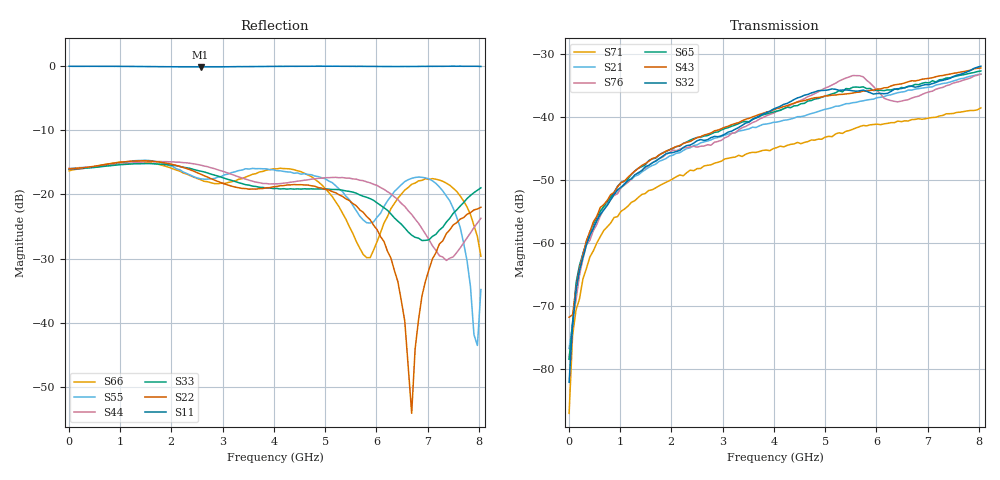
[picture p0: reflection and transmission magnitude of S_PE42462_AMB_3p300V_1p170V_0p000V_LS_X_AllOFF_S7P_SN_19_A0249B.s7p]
! Device ID: PE42462
! File Path: z:\PE42462\DataSheet S-parameter-6T\With_All_Off_States\Remeasure\AMB\3p300\LS_X\PE42462_AMB_3p300V_1p170V_0p000V_LS_X_AllOFF_S7P_SN_19_A0249B.s7p
! Serial: 19
! Lot: A0249B
! Temp: AMB
! VDD: 3.300
! VSS: 0.000
! Control_Hi: 1.170
! Control_Lo: 0.000
! Logic State: LS_X_AllOFF
! Port 1:
! Port 2:
! Port 3:
! Port 4:
! Port 5:
! Port 6:
! Port 7:
! ThroughPath:1-2
! IDD: 0.0001067802
! ISS/IDD2: -2.14e-008
! IDMM3/IDD3: -2.307e-007
! Comment:
#  Hz  S  RI  R  50
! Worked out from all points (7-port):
!   120 points, 10 MHz to 8.037 GHz, reference 50 ohm
!   strongest paths, dB at 10 MHz, 2.034 GHz, 4.057 GHz, 6.08 GHz, 8.037 GHz:
!     S32: -82.1, -45.7, -38.5, -36.3, -31.9
!     S43: -71.8, -44.9, -38.7, -35.5, -32.2
!     S65: -78.5, -45.0, -39.1, -35.8, -32.7
!     S76: -78.5, -45.3, -39.1, -36.3, -33.2
!     S21: -76.8, -46.1, -40.8, -36.9, -33.2
!     S71: -87.0, -49.8, -44.9, -41.2, -38.5
!   lowest |S11| = -0.2 dB at 2.573 GHz (marker M1), VSWR 112.77, Z = 0.444 - j2.34 ohm
!   |S11| at or under -10 dB: nowhere
